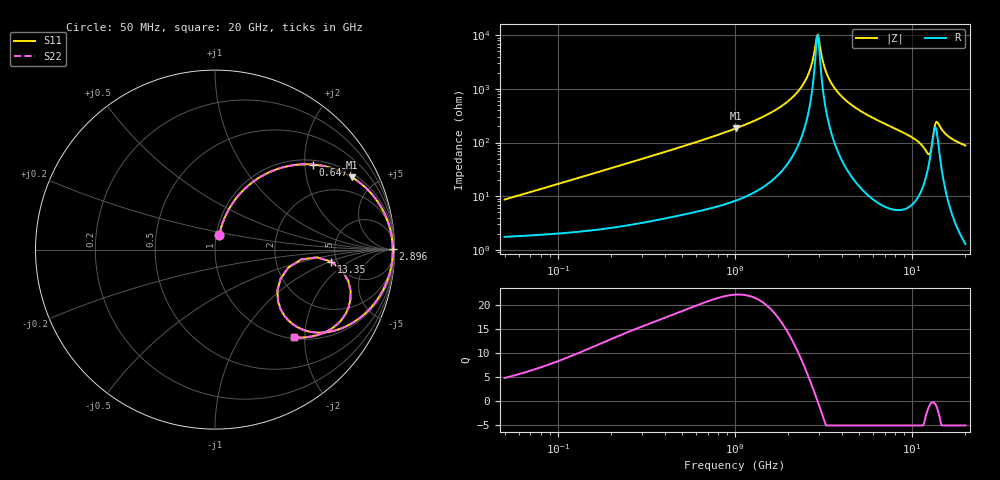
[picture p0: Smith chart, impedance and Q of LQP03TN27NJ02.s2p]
!Murata Part Number: LQP03TN27NJ02
!These Parameters are Measured in Series Mode Connection
!  o--[Z]--o
!Port1  Port2
!  o-------o
!Freq. Start=50[MHz] Stop=20[GHz], 401[Steps]
# Hz S RI R 50
!Freq.(Hz) S11(Real) S11(Imag) S21(Real) S21(Imag) S12(Real) S12(Imag) S22(Real) S22(Imag)
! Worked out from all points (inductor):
!   401 points, 50 MHz to 20 GHz, reference 50 ohm
!   read as one part in series: L = 27 nH near 51.52 MHz
!   highest Q = 22.2 at 1.015 GHz (marker M1), where L = 29 nH
!   self-resonance near 2.896 GHz
!   S11 on the Smith chart (normalised r, x): 50 MHz: 1.04, +0.17; 647.7 MHz: 1.11, +2.20; 2.896 GHz: open; 13.35 GHz: 4.49, -1.05; 20 GHz: 1.03, -1.76
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5e7  0.0241 0.0816  0.9759 -0.0816  0.9759 -0.0816  0.0241 0.0816
1.364002e8  0.0681 0.2081  0.9319 -0.2081  0.9319 -0.2081  0.0681 0.2081
3.721004e8  0.2886 0.4245  0.7114 -0.4245  0.7114 -0.4245  0.2886 0.4245
6.476653e8  0.5456 0.4739  0.4544 -0.4739  0.4544 -0.4739  0.5456 0.4739
1e9  0.7573 0.4067  0.2427 -0.4067  0.2427 -0.4067  0.7573 0.4067
1.015091e9  0.7638 0.4028  0.2362 -0.4028  0.2362 -0.4028  0.7638 0.4028
2.021818e9  0.9635 0.1549  0.0365 -0.1549  0.0365 -0.1549  0.9635 0.1549
2.456456e9  0.9842 0.0741  0.0158 -0.0741  0.0158 -0.0741  0.9842 0.0741
2.728004e9  0.9894 0.03  0.0106 -0.03  0.0106 -0.03  0.9894 0.03
2.896447e9  0.9905 0.00471  0.00952 -0.00471  0.00952 -0.00471  0.9905 0.00471
2.98453e9  0.9905 -0.00797  0.00946 0.00797  0.00946 0.00797  0.9905 -0.00797
3.314454e9  0.9881 -0.0525  0.0119 0.0525  0.0119 0.0525  0.9881 -0.0525
3.850025e9  0.9772 -0.1163  0.0228 0.1163  0.0228 0.1163  0.9772 -0.1163
4.966507e9  0.9367 -0.2248  0.0633 0.2248  0.0633 0.2248  0.9367 -0.2248
7.442007e9  0.7996 -0.3861  0.2004 0.3861  0.2004 0.3861  0.7996 -0.3861
1.066139e10  0.5363 -0.4589  0.4637 0.4589  0.4637 0.4589  0.5363 -0.4589
1.220001e10  0.3508 -0.2859  0.6492 0.2859  0.6492 0.2859  0.3508 -0.2859
1.276073e10  0.4086 -0.1002  0.5914 0.1002  0.5914 0.1002  0.4086 -0.1002
1.334722e10  0.6487 -0.0674  0.3513 0.0674  0.3513 0.0674  0.6487 -0.0674
1.417136e10  0.7543 -0.2799  0.2457 0.2799  0.2457 0.2799  0.7543 -0.2799
1.550395e10  0.6605 -0.4329  0.3395 0.4329  0.3395 0.4329  0.6605 -0.4329
2e10  0.4377 -0.4888  0.5623 0.4888  0.5623 0.4888  0.4377 -0.4888
